| / 7\'7   Xilinx Spartan-XL I/O Buffer IBIS File
| \ \   Xilinx Inc.
| / /   2100 Logic Drive
| \_\/.\   San Jose,   CA 95124
[IBIS ver]   2.1
[File name]   xcs00xl.ibs
[File Rev]   2.1
[Date]   June 17, 1999
[Source]   Spice netlist
[Notes]   - Best/worse process data included in this ibis model
   - Control flag setting:
   SLW=0 - fast slew rate
   SLW=1 - slow slew rate
   PCI=0 - driving 3.3V PCI bus, 12mA
   PCI=1 - driving 5.0V PCI bus, 24mA
   5VT=0 - 5.0V tolerant input off
   5VT=1 - 5.0V tolerant input on
   - Created by Joey Jia x4437
[Copyright]   Xilinx Inc. All right reserved
|   Component XCS05XL_PC84[SLW=0;PCI=0;5VT=0]
[Component]   XCS05XL_PC84[SLW=0;PCI=0;5VT=0]
[Manufacturer]   Xilinx Inc.
[Package]
| variable   typ   min   max
R_pkg   0.104   97.000m   0.111
L_pkg   11.600nH   10.200nH   13.000nH
C_pkg   1.700pF   1.600pF   1.800pF
[Pin]  signal_name   model_name   R_pin   L_pin   C_pin
io   iob   IO_000   NA   NA   NA
|   Component XCS05XL_PC84[SLW=0;PCI=0;5VT=1]
[Component]   XCS05XL_PC84[SLW=0;PCI=0;5VT=1]
[Manufacturer]   Xilinx Inc.
[Package]
| variable   typ   min   max
R_pkg   0.104   97.000m   0.111
L_pkg   11.600nH   10.200nH   13.000nH
C_pkg   1.700pF   1.600pF   1.800pF
[Pin]  signal_name   model_name   R_pin   L_pin   C_pin
io   iob   IO_001   NA   NA   NA
|   Component XCS05XL_PC84[SLW=0;PCI=1;5VT=0]
[Component]   XCS05XL_PC84[SLW=0;PCI=1;5VT=0]
[Manufacturer]   Xilinx Inc.
[Package]
| variable   typ   min   max
R_pkg   0.104   97.000m   0.111
L_pkg   11.600nH   10.200nH   13.000nH
C_pkg   1.700pF   1.600pF   1.800pF
[Pin]  signal_name   model_name   R_pin   L_pin   C_pin
io   iob   IO_010   NA   NA   NA
|   Component XCS05XL_PC84[SLW=0;PCI=1;5VT=1]
[Component]   XCS05XL_PC84[SLW=0;PCI=1;5VT=1]
[Manufacturer]   Xilinx Inc.
[Package]
| variable   typ   min   max
R_pkg   0.104   97.000m   0.111
L_pkg   11.600nH   10.200nH   13.000nH
C_pkg   1.700pF   1.600pF   1.800pF
[Pin]  signal_name   model_name   R_pin   L_pin   C_pin
io   iob   IO_011   NA   NA   NA
|   Component XCS05XL_PC84[SLW=1;PCI=0;5VT=0]
[Component]   XCS05XL_PC84[SLW=1;PCI=0;5VT=0]
[Manufacturer]   Xilinx Inc.
[Package]
| variable   typ   min   max
R_pkg   0.104   97.000m   0.111
L_pkg   11.600nH   10.200nH   13.000nH
C_pkg   1.700pF   1.600pF   1.800pF
[Pin]  signal_name   model_name   R_pin   L_pin   C_pin
io   iob   IO_100   NA   NA   NA
|   Component XCS05XL_PC84[SLW=1;PCI=0;5VT=1]
[Component]   XCS05XL_PC84[SLW=1;PCI=0;5VT=1]
[Manufacturer]   Xilinx Inc.
[Package]
| variable   typ   min   max
R_pkg   0.104   97.000m   0.111
L_pkg   11.600nH   10.200nH   13.000nH
C_pkg   1.700pF   1.600pF   1.800pF
[Pin]  signal_name   model_name   R_pin   L_pin   C_pin
io   iob   IO_101   NA   NA   NA
|   Component XCS05XL_PC84[SLW=1;PCI=1;5VT=0]
[Component]   XCS05XL_PC84[SLW=1;PCI=1;5VT=0]
[Manufacturer]   Xilinx Inc.
[Package]
| variable   typ   min   max
R_pkg   0.104   97.000m   0.111
L_pkg   11.600nH   10.200nH   13.000nH
C_pkg   1.700pF   1.600pF   1.800pF
[Pin]  signal_name   model_name   R_pin   L_pin   C_pin
io   iob   IO_110   NA   NA   NA
|   Component XCS05XL_PC84[SLW=1;PCI=1;5VT=1]
[Component]   XCS05XL_PC84[SLW=1;PCI=1;5VT=1]
[Manufacturer]   Xilinx Inc.
[Package]
| variable   typ   min   max
R_pkg   0.104   97.000m   0.111
L_pkg   11.600nH   10.200nH   13.000nH
C_pkg   1.700pF   1.600pF   1.800pF
[Pin]  signal_name   model_name   R_pin   L_pin   C_pin
io   iob   IO_111   NA   NA   NA
|+++++++++++++++++++++++++++++++++++++++++++++++++++++++++++++++++++++++++
|   Component XCS05XL_VQ100[SLW=0;PCI=0;5VT=0]
[Component]   XCS05XL_VQ100[SLW=0;PCI=0;5VT=0]
[Manufacturer]   Xilinx Inc.
[Package]
| variable   typ   min   max
R_pkg   101.500m   98.000m   105.000m
L_pkg   5.200nH   4.700nH   5.700nH
C_pkg   0.550pF   0.400pF   0.700pF
[Pin]  signal_name   model_name   R_pin   L_pin   C_pin
io   iob   IO_000   NA   NA   NA
| End [Component] XCS05XL_VQ100[SLW=0;PCI=0;5VT=0]
|   Component XCS05XL_VQ100[SLW=0;PCI=0;5VT=1]
[Component]   XCS05XL_VQ100[SLW=0;PCI=0;5VT=1]
[Manufacturer]   Xilinx Inc.
[Package]
| variable   typ   min   max
R_pkg   101.500m   98.000m   105.000m
L_pkg   5.200nH   4.700nH   5.700nH
C_pkg   0.550pF   0.400pF   0.700pF
[Pin]  signal_name   model_name   R_pin   L_pin   C_pin
io   iob   IO_001   NA   NA   NA
| End [Component] XCS05XL_VQ100[SLW=0;PCI=0;5VT=1]
|   Component XCS05XL_VQ100[SLW=0;PCI=1;5VT=0]
[Component]   XCS05XL_VQ100[SLW=0;PCI=1;5VT=0]
[Manufacturer]   Xilinx Inc.
[Package]
| variable   typ   min   max
R_pkg   101.500m   98.000m   105.000m
L_pkg   5.200nH   4.700nH   5.700nH
C_pkg   0.550pF   0.400pF   0.700pF
[Pin]  signal_name   model_name   R_pin   L_pin   C_pin
io   iob   IO_010   NA   NA   NA
| End [Component] XCS05XL_VQ100[SLW=0;PCI=1;5VT=0]
|   Component XCS05XL_VQ100[SLW=0;PCI=1;5VT=1]
[Component]   XCS05XL_VQ100[SLW=0;PCI=1;5VT=1]
[Manufacturer]   Xilinx Inc.
[Package]
| variable   typ   min   max
R_pkg   101.500m   98.000m   105.000m
L_pkg   5.200nH   4.700nH   5.700nH
C_pkg   0.550pF   0.400pF   0.700pF
[Pin]  signal_name   model_name   R_pin   L_pin   C_pin
io   iob   IO_011   NA   NA   NA
| End [Component] XCS05XL_VQ100[SLW=0;PCI=1;5VT=1]
|   Component XCS05XL_VQ100[SLW=1;PCI=0;5VT=0]
[Component]   XCS05XL_VQ100[SLW=1;PCI=0;5VT=0]
[Manufacturer]   Xilinx Inc.
[Package]
| variable   typ   min   max
R_pkg   101.500m   98.000m   105.000m
L_pkg   5.200nH   4.700nH   5.700nH
C_pkg   0.550pF   0.400pF   0.700pF
[Pin]  signal_name   model_name   R_pin   L_pin   C_pin
io   iob   IO_100   NA   NA   NA
| End [Component] XCS05XL_VQ100[SLW=1;PCI=0;5VT=0]
|   Component XCS05XL_VQ101[SLW=1;PCI=0;5VT=1]
[Component]   XCS05XL_VQ100[SLW=1;PCI=0;5VT=1]
[Manufacturer]   Xilinx Inc.
[Package]
| variable   typ   min   max
R_pkg   101.500m   98.000m   105.000m
L_pkg   5.200nH   4.700nH   5.700nH
C_pkg   0.550pF   0.400pF   0.700pF
[Pin]  signal_name   model_name   R_pin   L_pin   C_pin
io   iob   IO_101   NA   NA   NA
| End [Component] XCS05XL_VQ100[SLW=1;PCI=0;5VT=1]
|   Component XCS05XL_VQ100[SLW=1;PCI=1;5VT=0]
[Component]   XCS05XL_VQ100[SLW=1;PCI=1;5VT=0]
[Manufacturer]   Xilinx Inc.
[Package]
| variable   typ   min   max
R_pkg   101.500m   98.000m   105.000m
L_pkg   5.200nH   4.700nH   5.700nH
C_pkg   0.550pF   0.400pF   0.700pF
[Pin]  signal_name   model_name   R_pin   L_pin   C_pin
io   iob   IO_110   NA   NA   NA
| End [Component] XCS05XL_VQ100[SLW=1;PCI=1;5VT=0]
|   Component XCS05XL_VQ100[SLW=1;PCI=1;5VT=1]
[Component]   XCS05XL_VQ100[SLW=1;PCI=1;5VT=1]
[Manufacturer]   Xilinx Inc.
[Package]
| variable   typ   min   max
R_pkg   101.500m   98.000m   105.000m
L_pkg   5.200nH   4.700nH   5.700nH
C_pkg   0.550pF   0.400pF   0.700pF
[Pin]  signal_name   model_name   R_pin   L_pin   C_pin
io   iob   IO_111   NA   NA   NA
| End [Component] XCS05XL_VQ100[SLW=1;PCI=1;5VT=1]
|+++++++++++++++++++++++++++++++++++++++++++++++++++++++++++++++++++++++++
|   Component XCS10XL_PC84[SLW=0;PCI=0;5VT=0]
[Component]   XCS10XL_PC84[SLW=0;PCI=0;5VT=0]
[Manufacturer]   Xilinx Inc.
[Package]
| variable   typ   min   max
R_pkg   104.000m   97.000m   111.000m
L_pkg   11.600nH   10.200nH   13.000nH
C_pkg   1.700pF   1.600pF   1.800pF
[Pin]  signal_name   model_name   R_pin   L_pin   C_pin
io   iob   IO_000   NA   NA   NA
| End [Component] XCS10XL_PC84[SLW=0;PCI=0;5VT=0]
|   Component XCS10XL_PC84[SLW=0;PCI=0;5VT=1]
[Component]   XCS10XL_PC84[SLW=0;PCI=0;5VT=1]
[Manufacturer]   Xilinx Inc.
[Package]
| variable   typ   min   max
R_pkg   104.000m   97.000m   111.000m
L_pkg   11.600nH   10.200nH   13.000nH
C_pkg   1.700pF   1.600pF   1.800pF
[Pin]  signal_name   model_name   R_pin   L_pin   C_pin
io   iob   IO_001   NA   NA   NA
| End [Component] XCS10XL_PC84[SLW=0;PCI=0;5VT=1]
|   Component XCS10XL_PC84[SLW=0;PCI=1;5VT=0]
[Component]   XCS10XL_PC84[SLW=0;PCI=1;5VT=0]
[Manufacturer]   Xilinx Inc.
[Package]
| variable   typ   min   max
R_pkg   104.000m   97.000m   111.000m
L_pkg   11.600nH   10.200nH   13.000nH
C_pkg   1.700pF   1.600pF   1.800pF
[Pin]  signal_name   model_name   R_pin   L_pin   C_pin
io   iob   IO_010   NA   NA   NA
| End [Component] XCS10XL_PC84[SLW=0;PCI=1;5VT=0]
|   Component XCS10XL_PC84[SLW=0;PCI=1;5VT=1]
[Component]   XCS10XL_PC84[SLW=0;PCI=1;5VT=1]
[Manufacturer]   Xilinx Inc.
[Package]
| variable   typ   min   max
R_pkg   104.000m   97.000m   111.000m
L_pkg   11.600nH   10.200nH   13.000nH
C_pkg   1.700pF   1.600pF   1.800pF
[Pin]  signal_name   model_name   R_pin   L_pin   C_pin
io   iob   IO_011   NA   NA   NA
| End [Component] XCS10XL_PC84[SLW=0;PCI=1;5VT=1]
|   Component XCS10XL_PC84[SLW=1;PCI=0;5VT=0]
[Component]   XCS10XL_PC84[SLW=1;PCI=0;5VT=0]
[Manufacturer]   Xilinx Inc.
[Package]
| variable   typ   min   max
R_pkg   104.000m   97.000m   111.000m
L_pkg   11.600nH   10.200nH   13.000nH
C_pkg   1.700pF   1.600pF   1.800pF
[Pin]  signal_name   model_name   R_pin   L_pin   C_pin
io   iob   IO_100   NA   NA   NA
| End [Component] XCS10XL_PC84[SLW=1;PCI=0;5VT=0]
|   Component XCS10XL_PC84[SLW=1;PCI=0;5VT=1]
[Component]   XCS10XL_PC84[SLW=1;PCI=0;5VT=1]
[Manufacturer]   Xilinx Inc.
[Package]
| variable   typ   min   max
R_pkg   104.000m   97.000m   111.000m
L_pkg   11.600nH   10.200nH   13.000nH
C_pkg   1.700pF   1.600pF   1.800pF
[Pin]  signal_name   model_name   R_pin   L_pin   C_pin
io   iob   IO_101   NA   NA   NA
| End [Component] XCS10XL_PC84[SLW=1;PCI=0;5VT=1]
|   Component XCS10XL_PC84[SLW=1;PCI=1;5VT=0]
[Component]   XCS10XL_PC84[SLW=1;PCI=1;5VT=0]
[Manufacturer]   Xilinx Inc.
[Package]
| variable   typ   min   max
R_pkg   104.000m   97.000m   111.000m
L_pkg   11.600nH   10.200nH   13.000nH
C_pkg   1.700pF   1.600pF   1.800pF
[Pin]  signal_name   model_name   R_pin   L_pin   C_pin
io   iob   IO_110   NA   NA   NA
| End [Component] XCS10XL_PC84[SLW=1;PCI=1;5VT=0]
|   Component XCS10XL_PC84[SLW=1;PCI=1;5VT=1]
[Component]   XCS10XL_PC84[SLW=1;PCI=1;5VT=1]
[Manufacturer]   Xilinx Inc.
[Package]
| variable   typ   min   max
R_pkg   104.000m   97.000m   111.000m
L_pkg   11.600nH   10.200nH   13.000nH
C_pkg   1.700pF   1.600pF   1.800pF
[Pin]  signal_name   model_name   R_pin   L_pin   C_pin
io   iob   IO_111   NA   NA   NA
| End [Component] XCS10XL_PC84[SLW=1;PCI=1;5VT=1]
|+++++++++++++++++++++++++++++++++++++++++++++++++++++++++++++++++++++++++
|   Component XCS10XL_VQ100[SLW=0;PCI=0;5VT=0]
[Component]   XCS10XL_VQ100[SLW=0;PCI=0;5VT=0]
[Manufacturer]   Xilinx Inc.
[Package]
| variable   typ   min   max
R_pkg   101.500m   98.000m   105.000m
L_pkg   5.200nH   4.700nH   5.700nH
C_pkg   0.550pF   0.400pF   0.700pF
[Pin]  signal_name   model_name   R_pin   L_pin   C_pin
io   iob   IO_000   NA   NA   NA
| End [Component] XCS10XL_VQ100[SLW=0;PCI=0;5VT=0]
|   Component XCS10XL_VQ100[SLW=0;PCI=0;5VT=1]
[Component]   XCS10XL_VQ100[SLW=0;PCI=0;5VT=1]
[Manufacturer]   Xilinx Inc.
[Package]
| variable   typ   min   max
R_pkg   101.500m   98.000m   105.000m
L_pkg   5.200nH   4.700nH   5.700nH
C_pkg   0.550pF   0.400pF   0.700pF
[Pin]  signal_name   model_name   R_pin   L_pin   C_pin
io   iob   IO_001   NA   NA   NA
| End [Component] XCS10XL_VQ100[SLW=0;PCI=0;5VT=1]
|   Component XCS10XL_VQ100[SLW=0;PCI=1;5VT=0]
[Component]   XCS10XL_VQ100[SLW=0;PCI=1;5VT=0]
[Manufacturer]   Xilinx Inc.
[Package]
| variable   typ   min   max
R_pkg   101.500m   98.000m   105.000m
L_pkg   5.200nH   4.700nH   5.700nH
C_pkg   0.550pF   0.400pF   0.700pF
[Pin]  signal_name   model_name   R_pin   L_pin   C_pin
io   iob   IO_010   NA   NA   NA
| End [Component] XCS10XL_VQ100[SLW=0;PCI=1;5VT=0]
|   Component XCS10XL_VQ100[SLW=0;PCI=1;5VT=1]
[Component]   XCS10XL_VQ100[SLW=0;PCI=1;5VT=1]
[Manufacturer]   Xilinx Inc.
[Package]
| variable   typ   min   max
R_pkg   101.500m   98.000m   105.000m
L_pkg   5.200nH   4.700nH   5.700nH
C_pkg   0.550pF   0.400pF   0.700pF
[Pin]  signal_name   model_name   R_pin   L_pin   C_pin
io   iob   IO_011   NA   NA   NA
| End [Component] XCS10XL_VQ100[SLW=0;PCI=1;5VT=1]
|   Component XCS10XL_VQ100[SLW=1;PCI=0;5VT=0]
[Component]   XCS10XL_VQ100[SLW=1;PCI=0;5VT=0]
[Manufacturer]   Xilinx Inc.
[Package]
| variable   typ   min   max
R_pkg   101.500m   98.000m   105.000m
L_pkg   5.200nH   4.700nH   5.700nH
C_pkg   0.550pF   0.400pF   0.700pF
[Pin]  signal_name   model_name   R_pin   L_pin   C_pin
io   iob   IO_100   NA   NA   NA
| End [Component] XCS10XL_VQ100[SLW=1;PCI=0;5VT=0]
|   Component XCS10XL_VQ100[SLW=1;PCI=0;5VT=1]
[Component]   XCS10XL_VQ100[SLW=1;PCI=0;5VT=1]
[Manufacturer]   Xilinx Inc.
[Package]
| variable   typ   min   max
R_pkg   101.500m   98.000m   105.000m
L_pkg   5.200nH   4.700nH   5.700nH
C_pkg   0.550pF   0.400pF   0.700pF
[Pin]  signal_name   model_name   R_pin   L_pin   C_pin
io   iob   IO_101   NA   NA   NA
| End [Component] XCS10XL_VQ100[SLW=1;PCI=0;5VT=1]
|   Component XCS10XL_VQ100[SLW=1;PCI=1;5VT=0]
[Component]   XCS10XL_VQ100[SLW=1;PCI=1;5VT=0]
[Manufacturer]   Xilinx Inc.
[Package]
| variable   typ   min   max
R_pkg   101.500m   98.000m   105.000m
L_pkg   5.200nH   4.700nH   5.700nH
C_pkg   0.550pF   0.400pF   0.700pF
[Pin]  signal_name   model_name   R_pin   L_pin   C_pin
io   iob   IO_110   NA   NA   NA
| End [Component] XCS10XL_VQ100[SLW=1;PCI=1;5VT=0]
|   Component XCS10XL_VQ100[SLW=1;PCI=1;5VT=1]
[Component]   XCS10XL_VQ100[SLW=1;PCI=1;5VT=1]
[Manufacturer]   Xilinx Inc.
[Package]
| variable   typ   min   max
R_pkg   101.500m   98.000m   105.000m
L_pkg   5.200nH   4.700nH   5.700nH
C_pkg   0.550pF   0.400pF   0.700pF
[Pin]  signal_name   model_name   R_pin   L_pin   C_pin
io   iob   IO_111   NA   NA   NA
| End [Component] XCS10XL_VQ100[SLW=1;PCI=1;5VT=1]
|+++++++++++++++++++++++++++++++++++++++++++++++++++++++++++++++++++++++++
|   Component XCS10XL_TQ144[SLW=0;PCI=0;5VT=0]
[Component]   XCS10XL_TQ144[SLW=0;PCI=0;5VT=0]
[Manufacturer]   Xilinx Inc.
[Package]
| variable   typ   min   max
R_pkg   123.500m   117.000m   130.000m
L_pkg   7.950nH   7.100nH   8.800nH
C_pkg   1.000pF   0.800pF   1.200pF
[Pin]  signal_name   model_name   R_pin   L_pin   C_pin
io   iob   IO_000   NA   NA   NA
| End [Component] XCS10XL_TQ144[SLW=0;PCI=0;5VT=0]
|   Component XCS10XL_TQ144[SLW=0;PCI=0;5VT=1]
[Component]   XCS10XL_TQ144[SLW=0;PCI=0;5VT=1]
[Manufacturer]   Xilinx Inc.
[Package]
| variable   typ   min   max
R_pkg   123.500m   117.000m   130.000m
L_pkg   7.950nH   7.100nH   8.800nH
C_pkg   1.000pF   0.800pF   1.200pF
[Pin]  signal_name   model_name   R_pin   L_pin   C_pin
io   iob   IO_001   NA   NA   NA
| End [Component] XCS10XL_TQ144[SLW=0;PCI=0;5VT=1]
|   Component XCS10XL_TQ144[SLW=0;PCI=1;5VT=0]
[Component]   XCS10XL_TQ144[SLW=0;PCI=1;5VT=0]
[Manufacturer]   Xilinx Inc.
[Package]
| variable   typ   min   max
R_pkg   123.500m   117.000m   130.000m
L_pkg   7.950nH   7.100nH   8.800nH
C_pkg   1.000pF   0.800pF   1.200pF
[Pin]  signal_name   model_name   R_pin   L_pin   C_pin
io   iob   IO_010   NA   NA   NA
| End [Component] XCS10XL_TQ144[SLW=0;PCI=1;5VT=0]
|   Component XCS10XL_TQ144[SLW=0;PCI=1;5VT=1]
[Component]   XCS10XL_TQ144[SLW=0;PCI=1;5VT=1]
[Manufacturer]   Xilinx Inc.
[Package]
| variable   typ   min   max
R_pkg   123.500m   117.000m   130.000m
L_pkg   7.950nH   7.100nH   8.800nH
C_pkg   1.000pF   0.800pF   1.200pF
[Pin]  signal_name   model_name   R_pin   L_pin   C_pin
io   iob   IO_011   NA   NA   NA
| End [Component] XCS10XL_TQ144[SLW=0;PCI=1;5VT=1]
|   Component XCS10XL_TQ144[SLW=1;PCI=0;5VT=0]
[Component]   XCS10XL_TQ144[SLW=1;PCI=0;5VT=0]
[Manufacturer]   Xilinx Inc.
[Package]
| variable   typ   min   max
R_pkg   123.500m   117.000m   130.000m
L_pkg   7.950nH   7.100nH   8.800nH
C_pkg   1.000pF   0.800pF   1.200pF
[Pin]  signal_name   model_name   R_pin   L_pin   C_pin
io   iob   IO_100   NA   NA   NA
| End [Component] XCS10XL_TQ144[SLW=1;PCI=0;5VT=0]
|   Component XCS10XL_TQ144[SLW=1;PCI=0;5VT=1]
[Component]   XCS10XL_TQ144[SLW=1;PCI=0;5VT=1]
[Manufacturer]   Xilinx Inc.
[Package]
| variable   typ   min   max
R_pkg   123.500m   117.000m   130.000m
L_pkg   7.950nH   7.100nH   8.800nH
C_pkg   1.000pF   0.800pF   1.200pF
[Pin]  signal_name   model_name   R_pin   L_pin   C_pin
io   iob   IO_101   NA   NA   NA
| End [Component] XCS10XL_TQ144[SLW=1;PCI=0;5VT=1]
|   Component XCS10XL_TQ144[SLW=1;PCI=1;5VT=0]
[Component]   XCS10XL_TQ144[SLW=1;PCI=1;5VT=0]
[Manufacturer]   Xilinx Inc.
[Package]
| variable   typ   min   max
R_pkg   123.500m   117.000m   130.000m
L_pkg   7.950nH   7.100nH   8.800nH
C_pkg   1.000pF   0.800pF   1.200pF
[Pin]  signal_name   model_name   R_pin   L_pin   C_pin
io   iob   IO_110   NA   NA   NA
| End [Component] XCS10XL_TQ144[SLW=1;PCI=1;5VT=0]
|   Component XCS10XL_TQ144[SLW=1;PCI=1;5VT=1]
[Component]   XCS10XL_TQ144[SLW=1;PCI=1;5VT=1]
[Manufacturer]   Xilinx Inc.
[Package]
| variable   typ   min   max
R_pkg   123.500m   117.000m   130.000m
L_pkg   7.950nH   7.100nH   8.800nH
C_pkg   1.000pF   0.800pF   1.200pF
[Pin]  signal_name   model_name   R_pin   L_pin   C_pin
io   iob   IO_111   NA   NA   NA
| End [Component] XCS10XL_TQ144[SLW=1;PCI=1;5VT=1]
|+++++++++++++++++++++++++++++++++++++++++++++++++++++++++++++++++++++++++
|   Component XCS20XL_VQ100[SLW=0;PCI=0;5VT=0]
[Component]   XCS20XL_VQ100[SLW=0;PCI=0;5VT=0]
[Manufacturer]   Xilinx Inc.
[Package]
| variable   typ   min   max
R_pkg   101.500m   98.000m   105.000m
L_pkg   5.200nH   4.700nH   5.700nH
C_pkg   0.550pF   0.400pF   0.700pF
[Pin]  signal_name   model_name   R_pin   L_pin   C_pin
io   iob   IO_000   NA   NA   NA
| End [Component] XCS20XL_VQ100[SLW=0;PCI=0;5VT=0]
|   Component XCS20XL_VQ100[SLW=0;PCI=0;5VT=1]
[Component]   XCS20XL_VQ100[SLW=0;PCI=0;5VT=1]
[Manufacturer]   Xilinx Inc.
[Package]
| variable   typ   min   max
R_pkg   101.500m   98.000m   105.000m
L_pkg   5.200nH   4.700nH   5.700nH
C_pkg   0.550pF   0.400pF   0.700pF
[Pin]  signal_name   model_name   R_pin   L_pin   C_pin
io   iob   IO_001   NA   NA   NA
| End [Component] XCS20XL_VQ100[SLW=0;PCI=0;5VT=1]
|   Component XCS20XL_VQ100[SLW=0;PCI=1;5VT=0]
[Component]   XCS20XL_VQ100[SLW=0;PCI=1;5VT=0]
[Manufacturer]   Xilinx Inc.
[Package]
| variable   typ   min   max
R_pkg   101.500m   98.000m   105.000m
L_pkg   5.200nH   4.700nH   5.700nH
C_pkg   0.550pF   0.400pF   0.700pF
[Pin]  signal_name   model_name   R_pin   L_pin   C_pin
io   iob   IO_010   NA   NA   NA
| End [Component] XCS20XL_VQ100[SLW=0;PCI=1;5VT=0]
|   Component XCS20XL_VQ100[SLW=0;PCI=1;5VT=1]
[Component]   XCS20XL_VQ100[SLW=0;PCI=1;5VT=1]
[Manufacturer]   Xilinx Inc.
[Package]
| variable   typ   min   max
R_pkg   101.500m   98.000m   105.000m
L_pkg   5.200nH   4.700nH   5.700nH
C_pkg   0.550pF   0.400pF   0.700pF
[Pin]  signal_name   model_name   R_pin   L_pin   C_pin
io   iob   IO_011   NA   NA   NA
| End [Component] XCS20XL_VQ100[SLW=0;PCI=1;5VT=1]
|   Component XCS20XL_VQ100[SLW=1;PCI=0;5VT=0]
[Component]   XCS20XL_VQ100[SLW=1;PCI=0;5VT=0]
[Manufacturer]   Xilinx Inc.
[Package]
| variable   typ   min   max
R_pkg   101.500m   98.000m   105.000m
L_pkg   5.200nH   4.700nH   5.700nH
C_pkg   0.550pF   0.400pF   0.700pF
[Pin]  signal_name   model_name   R_pin   L_pin   C_pin
io   iob   IO_100   NA   NA   NA
| End [Component] XCS20XL_VQ100[SLW=1;PCI=0;5VT=0]
|   Component XCS20XL_VQ100[SLW=1;PCI=0;5VT=1]
[Component]   XCS20XL_VQ100[SLW=1;PCI=0;5VT=1]
[Manufacturer]   Xilinx Inc.
[Package]
| variable   typ   min   max
R_pkg   101.500m   98.000m   105.000m
L_pkg   5.200nH   4.700nH   5.700nH
C_pkg   0.550pF   0.400pF   0.700pF
[Pin]  signal_name   model_name   R_pin   L_pin   C_pin
io   iob   IO_101   NA   NA   NA
| End [Component] XCS20XL_VQ100[SLW=1;PCI=0;5VT=1]
|   Component XCS20XL_VQ100[SLW=1;PCI=1;5VT=0]
[Component]   XCS20XL_VQ100[SLW=1;PCI=1;5VT=0]
[Manufacturer]   Xilinx Inc.
[Package]
| variable   typ   min   max
R_pkg   101.500m   98.000m   105.000m
L_pkg   5.200nH   4.700nH   5.700nH
C_pkg   0.550pF   0.400pF   0.700pF
[Pin]  signal_name   model_name   R_pin   L_pin   C_pin
io   iob   IO_110   NA   NA   NA
| End [Component] XCS20XL_VQ100[SLW=1;PCI=1;5VT=0]
|   Component XCS20XL_VQ100[SLW=1;PCI=1;5VT=1]
[Component]   XCS20XL_VQ100[SLW=1;PCI=1;5VT=1]
[Manufacturer]   Xilinx Inc.
[Package]
| variable   typ   min   max
R_pkg   101.500m   98.000m   105.000m
L_pkg   5.200nH   4.700nH   5.700nH
C_pkg   0.550pF   0.400pF   0.700pF
[Pin]  signal_name   model_name   R_pin   L_pin   C_pin
io   iob   IO_111   NA   NA   NA
| End [Component] XCS20XL_VQ100[SLW=1;PCI=1;5VT=1]
|+++++++++++++++++++++++++++++++++++++++++++++++++++++++++++++++++++++++++
|   Component XCS20XL_TQ144[SLW=0;PCI=0;5VT=0]
[Component]   XCS20XL_TQ144[SLW=0;PCI=0;5VT=0]
[Manufacturer]   Xilinx Inc.
[Package]
| variable   typ   min   max
R_pkg   123.500m   117.000m   130.000m
L_pkg   7.950nH   7.100nH   8.800nH
C_pkg   1.000pF   0.800pF   1.200pF
[Pin]  signal_name   model_name   R_pin   L_pin   C_pin
io   iob   IO_000   NA   NA   NA
| End [Component] XCS20XL_TQ144[SLW=0;PCI=0;5VT=0]
|   Component XCS20XL_TQ144[SLW=0;PCI=0;5VT=1]
[Component]   XCS20XL_TQ144[SLW=0;PCI=0;5VT=1]
[Manufacturer]   Xilinx Inc.
[Package]
| variable   typ   min   max
R_pkg   123.500m   117.000m   130.000m
L_pkg   7.950nH   7.100nH   8.800nH
C_pkg   1.000pF   0.800pF   1.200pF
[Pin]  signal_name   model_name   R_pin   L_pin   C_pin
io   iob   IO_001   NA   NA   NA
| End [Component] XCS20XL_TQ144[SLW=0;PCI=0;5VT=1]
|   Component XCS20XL_TQ144[SLW=0;PCI=1;5VT=0]
[Component]   XCS20XL_TQ144[SLW=0;PCI=1;5VT=0]
[Manufacturer]   Xilinx Inc.
[Package]
| variable   typ   min   max
R_pkg   123.500m   117.000m   130.000m
L_pkg   7.950nH   7.100nH   8.800nH
C_pkg   1.000pF   0.800pF   1.200pF
[Pin]  signal_name   model_name   R_pin   L_pin   C_pin
io   iob   IO_010   NA   NA   NA
| End [Component] XCS20XL_TQ144[SLW=0;PCI=1;5VT=0]
|   Component XCS20XL_TQ144[SLW=0;PCI=1;5VT=1]
[Component]   XCS20XL_TQ144[SLW=0;PCI=1;5VT=1]
[Manufacturer]   Xilinx Inc.
[Package]
| variable   typ   min   max
R_pkg   123.500m   117.000m   130.000m
L_pkg   7.950nH   7.100nH   8.800nH
C_pkg   1.000pF   0.800pF   1.200pF
[Pin]  signal_name   model_name   R_pin   L_pin   C_pin
io   iob   IO_011   NA   NA   NA
| End [Component] XCS20XL_TQ144[SLW=0;PCI=1;5VT=1]
|   Component XCS20XL_TQ144[SLW=1;PCI=0;5VT=0]
[Component]   XCS20XL_TQ144[SLW=1;PCI=0;5VT=0]
[Manufacturer]   Xilinx Inc.
[Package]
| variable   typ   min   max
R_pkg   123.500m   117.000m   130.000m
L_pkg   7.950nH   7.100nH   8.800nH
C_pkg   1.000pF   0.800pF   1.200pF
[Pin]  signal_name   model_name   R_pin   L_pin   C_pin
io   iob   IO_100   NA   NA   NA
| End [Component] XCS20XL_TQ144[SLW=1;PCI=0;5VT=0]
|   Component XCS20XL_TQ144[SLW=1;PCI=0;5VT=1]
[Component]   XCS20XL_TQ144[SLW=1;PCI=0;5VT=1]
[Manufacturer]   Xilinx Inc.
[Package]
| variable   typ   min   max
R_pkg   123.500m   117.000m   130.000m
L_pkg   7.950nH   7.100nH   8.800nH
C_pkg   1.000pF   0.800pF   1.200pF
[Pin]  signal_name   model_name   R_pin   L_pin   C_pin
io   iob   IO_101   NA   NA   NA
| End [Component] XCS20XL_TQ144[SLW=1;PCI=0;5VT=1]
|   Component XCS20XL_TQ144[SLW=1;PCI=1;5VT=0]
[Component]   XCS20XL_TQ144[SLW=1;PCI=1;5VT=0]
[Manufacturer]   Xilinx Inc.
[Package]
| variable   typ   min   max
R_pkg   123.500m   117.000m   130.000m
L_pkg   7.950nH   7.100nH   8.800nH
C_pkg   1.000pF   0.800pF   1.200pF
[Pin]  signal_name   model_name   R_pin   L_pin   C_pin
io   iob   IO_110   NA   NA   NA
| End [Component] XCS20XL_TQ144[SLW=1;PCI=1;5VT=0]
|   Component XCS20XL_TQ144[SLW=1;PCI=1;5VT=1]
[Component]   XCS20XL_TQ144[SLW=1;PCI=1;5VT=1]
[Manufacturer]   Xilinx Inc.
[Package]
| variable   typ   min   max
R_pkg   123.500m   117.000m   130.000m
L_pkg   7.950nH   7.100nH   8.800nH
C_pkg   1.000pF   0.800pF   1.200pF
[Pin]  signal_name   model_name   R_pin   L_pin   C_pin
io   iob   IO_111   NA   NA   NA
| End [Component] XCS20XL_TQ144[SLW=1;PCI=1;5VT=1]
|+++++++++++++++++++++++++++++++++++++++++++++++++++++++++++++++++++++++++
|   Component XCS20XL_PQ208[SLW=0;PCI=0;5VT=0]
[Component]   XCS20XL_PQ208[SLW=0;PCI=0;5VT=0]
[Manufacturer]   Xilinx Inc.
[Package]
| variable   typ   min   max
R_pkg   195.500m   195.000m   196.000m
L_pkg   14.200nH   12.500nH   15.900nH
C_pkg   1.800pF   1.600pF   2.000pF
[Pin]  signal_name   model_name   R_pin   L_pin   C_pin
io   iob   IO_000   NA   NA   NA
| End [Component] XCS20XL_PQ208[SLW=0;PCI=0;5VT=0]
|   Component XCS20XL_PQ208[SLW=0;PCI=0;5VT=1]
[Component]   XCS20XL_PQ208[SLW=0;PCI=0;5VT=1]
[Manufacturer]   Xilinx Inc.
[Package]
| variable   typ   min   max
R_pkg   195.500m   195.000m   196.000m
L_pkg   14.200nH   12.500nH   15.900nH
C_pkg   1.800pF   1.600pF   2.000pF
[Pin]  signal_name   model_name   R_pin   L_pin   C_pin
io   iob   IO_001   NA   NA   NA
| End [Component] XCS20XL_PQ208[SLW=0;PCI=0;5VT=1]
|   Component XCS20XL_PQ208[SLW=0;PCI=1;5VT=0]
[Component]   XCS20XL_PQ208[SLW=0;PCI=1;5VT=0]
[Manufacturer]   Xilinx Inc.
[Package]
| variable   typ   min   max
R_pkg   195.500m   195.000m   196.000m
L_pkg   14.200nH   12.500nH   15.900nH
C_pkg   1.800pF   1.600pF   2.000pF
[Pin]  signal_name   model_name   R_pin   L_pin   C_pin
io   iob   IO_010   NA   NA   NA
| End [Component] XCS20XL_PQ208[SLW=0;PCI=1;5VT=0]
|   Component XCS20XL_PQ208[SLW=0;PCI=1;5VT=1]
[Component]   XCS20XL_PQ208[SLW=0;PCI=1;5VT=1]
[Manufacturer]   Xilinx Inc.
[Package]
| variable   typ   min   max
R_pkg   195.500m   195.000m   196.000m
L_pkg   14.200nH   12.500nH   15.900nH
C_pkg   1.800pF   1.600pF   2.000pF
[Pin]  signal_name   model_name   R_pin   L_pin   C_pin
io   iob   IO_011   NA   NA   NA
| End [Component] XCS20XL_PQ208[SLW=0;PCI=1;5VT=1]
|   Component XCS20XL_PQ208[SLW=1;PCI=0;5VT=0]
[Component]   XCS20XL_PQ208[SLW=1;PCI=0;5VT=0]
[Manufacturer]   Xilinx Inc.
[Package]
| variable   typ   min   max
R_pkg   195.500m   195.000m   196.000m
L_pkg   14.200nH   12.500nH   15.900nH
C_pkg   1.800pF   1.600pF   2.000pF
[Pin]  signal_name   model_name   R_pin   L_pin   C_pin
io   iob   IO_100   NA   NA   NA
| End [Component] XCS20XL_PQ208[SLW=1;PCI=0;5VT=0]
|   Component XCS20XL_PQ208[SLW=1;PCI=0;5VT=1]
[Component]   XCS20XL_PQ208[SLW=1;PCI=0;5VT=1]
[Manufacturer]   Xilinx Inc.
[Package]
| variable   typ   min   max
R_pkg   195.500m   195.000m   196.000m
L_pkg   14.200nH   12.500nH   15.900nH
C_pkg   1.800pF   1.600pF   2.000pF
[Pin]  signal_name   model_name   R_pin   L_pin   C_pin
io   iob   IO_101   NA   NA   NA
| End [Component] XCS20XL_PQ208[SLW=1;PCI=0;5VT=1]
|   Component XCS20XL_PQ208[SLW=1;PCI=1;5VT=0]
[Component]   XCS20XL_PQ208[SLW=1;PCI=1;5VT=0]
[Manufacturer]   Xilinx Inc.
[Package]
| variable   typ   min   max
R_pkg   195.500m   195.000m   196.000m
L_pkg   14.200nH   12.500nH   15.900nH
C_pkg   1.800pF   1.600pF   2.000pF
[Pin]  signal_name   model_name   R_pin   L_pin   C_pin
io   iob   IO_110   NA   NA   NA
| End [Component] XCS20XL_PQ208[SLW=1;PCI=1;5VT=0]
|   Component XCS20XL_PQ208[SLW=1;PCI=1;5VT=1]
[Component]   XCS20XL_PQ208[SLW=1;PCI=1;5VT=1]
[Manufacturer]   Xilinx Inc.
[Package]
| variable   typ   min   max
R_pkg   195.500m   195.000m   196.000m
L_pkg   14.200nH   12.500nH   15.900nH
C_pkg   1.800pF   1.600pF   2.000pF
[Pin]  signal_name   model_name   R_pin   L_pin   C_pin
io   iob   IO_111   NA   NA   NA
| End [Component] XCS20XL_PQ208[SLW=1;PCI=1;5VT=1]
|+++++++++++++++++++++++++++++++++++++++++++++++++++++++++++++++++++++++++
|   Component XCS30XL_VQ100[SLW=0;PCI=0;5VT=0]
[Component]   XCS30XL_VQ100[SLW=0;PCI=0;5VT=0]
[Manufacturer]   Xilinx Inc.
[Package]
| variable   typ   min   max
R_pkg   84.500m   79.000m   90.000m
L_pkg   4.350nH   3.800nH   4.900nH
C_pkg   0.650pF   0.600pF   0.700pF
[Pin]  signal_name   model_name   R_pin   L_pin   C_pin
io   iob   IO_000   NA   NA   NA
| End [Component] XCS30XL_VQ100[SLW=0;PCI=0;5VT=0]
|   Component XCS30XL_VQ100[SLW=0;PCI=0;5VT=1]
[Component]   XCS30XL_VQ100[SLW=0;PCI=0;5VT=1]
[Manufacturer]   Xilinx Inc.
[Package]
| variable   typ   min   max
R_pkg   84.500m   79.000m   90.000m
L_pkg   4.350nH   3.800nH   4.900nH
C_pkg   0.650pF   0.600pF   0.700pF
[Pin]  signal_name   model_name   R_pin   L_pin   C_pin
io   iob   IO_001   NA   NA   NA
| End [Component] XCS30XL_VQ100[SLW=0;PCI=0;5VT=1]
|   Component XCS30XL_VQ100[SLW=0;PCI=1;5VT=0]
[Component]   XCS30XL_VQ100[SLW=0;PCI=1;5VT=0]
[Manufacturer]   Xilinx Inc.
[Package]
| variable   typ   min   max
R_pkg   84.500m   79.000m   90.000m
L_pkg   4.350nH   3.800nH   4.900nH
C_pkg   0.650pF   0.600pF   0.700pF
[Pin]  signal_name   model_name   R_pin   L_pin   C_pin
io   iob   IO_010   NA   NA   NA
| End [Component] XCS30XL_VQ100[SLW=0;PCI=1;5VT=0]
|   Component XCS30XL_VQ100[SLW=0;PCI=1;5VT=1]
[Component]   XCS30XL_VQ100[SLW=0;PCI=1;5VT=1]
[Manufacturer]   Xilinx Inc.
[Package]
| variable   typ   min   max
R_pkg   84.500m   79.000m   90.000m
L_pkg   4.350nH   3.800nH   4.900nH
C_pkg   0.650pF   0.600pF   0.700pF
[Pin]  signal_name   model_name   R_pin   L_pin   C_pin
io   iob   IO_011   NA   NA   NA
| End [Component] XCS30XL_VQ100[SLW=0;PCI=1;5VT=1]
|   Component XCS30XL_VQ100[SLW=1;PCI=0;5VT=0]
[Component]   XCS30XL_VQ100[SLW=1;PCI=0;5VT=0]
[Manufacturer]   Xilinx Inc.
[Package]
| variable   typ   min   max
R_pkg   84.500m   79.000m   90.000m
L_pkg   4.350nH   3.800nH   4.900nH
C_pkg   0.650pF   0.600pF   0.700pF
[Pin]  signal_name   model_name   R_pin   L_pin   C_pin
io   iob   IO_100   NA   NA   NA
| End [Component] XCS30XL_VQ100[SLW=1;PCI=0;5VT=0]
|   Component XCS30XL_VQ100[SLW=1;PCI=0;5VT=1]
[Component]   XCS30XL_VQ100[SLW=1;PCI=0;5VT=1]
[Manufacturer]   Xilinx Inc.
[Package]
| variable   typ   min   max
R_pkg   84.500m   79.000m   90.000m
L_pkg   4.350nH   3.800nH   4.900nH
C_pkg   0.650pF   0.600pF   0.700pF
[Pin]  signal_name   model_name   R_pin   L_pin   C_pin
io   iob   IO_101   NA   NA   NA
| End [Component] XCS30XL_VQ100[SLW=1;PCI=0;5VT=1]
|   Component XCS30XL_VQ100[SLW=1;PCI=1;5VT=0]
[Component]   XCS30XL_VQ100[SLW=1;PCI=1;5VT=0]
[Manufacturer]   Xilinx Inc.
[Package]
| variable   typ   min   max
R_pkg   84.500m   79.000m   90.000m
L_pkg   4.350nH   3.800nH   4.900nH
C_pkg   0.650pF   0.600pF   0.700pF
[Pin]  signal_name   model_name   R_pin   L_pin   C_pin
io   iob   IO_110   NA   NA   NA
| End [Component] XCS30XL_VQ100[SLW=1;PCI=1;5VT=0]
|   Component XCS30XL_VQ100[SLW=1;PCI=1;5VT=1]
[Component]   XCS30XL_VQ100[SLW=1;PCI=1;5VT=1]
[Manufacturer]   Xilinx Inc.
[Package]
| variable   typ   min   max
R_pkg   84.500m   79.000m   90.000m
L_pkg   4.350nH   3.800nH   4.900nH
C_pkg   0.650pF   0.600pF   0.700pF
[Pin]  signal_name   model_name   R_pin   L_pin   C_pin
io   iob   IO_111   NA   NA   NA
| End [Component] XCS30XL_VQ100[SLW=1;PCI=1;5VT=1]
|+++++++++++++++++++++++++++++++++++++++++++++++++++++++++++++++++++++++++
|   Component XCS30XL_TQ144[SLW=0;PCI=0;5VT=0]
[Component]   XCS30XL_TQ144[SLW=0;PCI=0;5VT=0]
[Manufacturer]   Xilinx Inc.
[Package]
| variable   typ   min   max
R_pkg   123.500m   117.000m   130.000m
L_pkg   7.950nH   7.100nH   8.800nH
C_pkg   1.000pF   0.800pF   1.200pF
[Pin]  signal_name   model_name   R_pin   L_pin   C_pin
io   iob   IO_000   NA   NA   NA
| End [Component] XCS30XL_TQ144[SLW=0;PCI=0;5VT=0]
|   Component XCS30XL_TQ144[SLW=0;PCI=0;5VT=1]
[Component]   XCS30XL_TQ144[SLW=0;PCI=0;5VT=1]
[Manufacturer]   Xilinx Inc.
[Package]
| variable   typ   min   max
R_pkg   123.500m   117.000m   130.000m
L_pkg   7.950nH   7.100nH   8.800nH
C_pkg   1.000pF   0.800pF   1.200pF
[Pin]  signal_name   model_name   R_pin   L_pin   C_pin
io   iob   IO_001   NA   NA   NA
| End [Component] XCS30XL_TQ144[SLW=0;PCI=0;5VT=1]
|   Component XCS30XL_TQ144[SLW=0;PCI=1;5VT=0]
[Component]   XCS30XL_TQ144[SLW=0;PCI=1;5VT=0]
[Manufacturer]   Xilinx Inc.
[Package]
| variable   typ   min   max
R_pkg   123.500m   117.000m   130.000m
L_pkg   7.950nH   7.100nH   8.800nH
C_pkg   1.000pF   0.800pF   1.200pF
[Pin]  signal_name   model_name   R_pin   L_pin   C_pin
io   iob   IO_010   NA   NA   NA
| End [Component] XCS30XL_TQ144[SLW=0;PCI=1;5VT=0]
|   Component XCS30XL_TQ144[SLW=0;PCI=1;5VT=1]
[Component]   XCS30XL_TQ144[SLW=0;PCI=1;5VT=1]
[Manufacturer]   Xilinx Inc.
[Package]
| variable   typ   min   max
R_pkg   123.500m   117.000m   130.000m
L_pkg   7.950nH   7.100nH   8.800nH
C_pkg   1.000pF   0.800pF   1.200pF
[Pin]  signal_name   model_name   R_pin   L_pin   C_pin
io   iob   IO_011   NA   NA   NA
| End [Component] XCS30XL_TQ144[SLW=0;PCI=1;5VT=1]
|   Component XCS30XL_TQ144[SLW=1;PCI=0;5VT=0]
[Component]   XCS30XL_TQ144[SLW=1;PCI=0;5VT=0]
[Manufacturer]   Xilinx Inc.
[Package]
| variable   typ   min   max
R_pkg   123.500m   117.000m   130.000m
L_pkg   7.950nH   7.100nH   8.800nH
C_pkg   1.000pF   0.800pF   1.200pF
[Pin]  signal_name   model_name   R_pin   L_pin   C_pin
io   iob   IO_100   NA   NA   NA
| End [Component] XCS30XL_TQ144[SLW=1;PCI=0;5VT=0]
|   Component XCS30XL_TQ144[SLW=1;PCI=0;5VT=1]
[Component]   XCS30XL_TQ144[SLW=1;PCI=0;5VT=1]
[Manufacturer]   Xilinx Inc.
[Package]
| variable   typ   min   max
R_pkg   123.500m   117.000m   130.000m
L_pkg   7.950nH   7.100nH   8.800nH
C_pkg   1.000pF   0.800pF   1.200pF
[Pin]  signal_name   model_name   R_pin   L_pin   C_pin
io   iob   IO_101   NA   NA   NA
| End [Component] XCS30XL_TQ144[SLW=1;PCI=0;5VT=1]
|   Component XCS30XL_TQ144[SLW=1;PCI=1;5VT=0]
[Component]   XCS30XL_TQ144[SLW=1;PCI=1;5VT=0]
[Manufacturer]   Xilinx Inc.
[Package]
| variable   typ   min   max
R_pkg   123.500m   117.000m   130.000m
L_pkg   7.950nH   7.100nH   8.800nH
C_pkg   1.000pF   0.800pF   1.200pF
[Pin]  signal_name   model_name   R_pin   L_pin   C_pin
io   iob   IO_110   NA   NA   NA
| End [Component] XCS30XL_TQ144[SLW=1;PCI=1;5VT=0]
|   Component XCS30XL_TQ144[SLW=1;PCI=1;5VT=1]
[Component]   XCS30XL_TQ144[SLW=1;PCI=1;5VT=1]
[Manufacturer]   Xilinx Inc.
[Package]
| variable   typ   min   max
R_pkg   123.500m   117.000m   130.000m
L_pkg   7.950nH   7.100nH   8.800nH
C_pkg   1.000pF   0.800pF   1.200pF
[Pin]  signal_name   model_name   R_pin   L_pin   C_pin
io   iob   IO_111   NA   NA   NA
| End [Component] XCS30XL_TQ144[SLW=1;PCI=1;5VT=1]
|+++++++++++++++++++++++++++++++++++++++++++++++++++++++++++++++++++++++++
|   Component XCS30XL_PQ208[SLW=0;PCI=0;5VT=0]
[Component]   XCS30XL_PQ208[SLW=0;PCI=0;5VT=0]
[Manufacturer]   Xilinx Inc.
[Package]
| variable   typ   min   max
R_pkg   195.500m   195.000m   196.000m
L_pkg   14.200nH   12.500nH   15.900nH
C_pkg   1.800pF   1.600pF   2.000pF
[Pin]  signal_name   model_name   R_pin   L_pin   C_pin
io   iob   IO_000   NA   NA   NA
| End [Component] XCS30XL_PQ208[SLW=0;PCI=0;5VT=0]
|   Component XCS30XL_PQ208[SLW=0;PCI=0;5VT=1]
[Component]   XCS30XL_PQ208[SLW=0;PCI=0;5VT=1]
[Manufacturer]   Xilinx Inc.
[Package]
| variable   typ   min   max
R_pkg   195.500m   195.000m   196.000m
L_pkg   14.200nH   12.500nH   15.900nH
C_pkg   1.800pF   1.600pF   2.000pF
[Pin]  signal_name   model_name   R_pin   L_pin   C_pin
io   iob   IO_001   NA   NA   NA
| End [Component] XCS30XL_PQ208[SLW=0;PCI=0;5VT=1]
|   Component XCS30XL_PQ208[SLW=0;PCI=1;5VT=0]
[Component]   XCS30XL_PQ208[SLW=0;PCI=1;5VT=0]
[Manufacturer]   Xilinx Inc.
[Package]
| variable   typ   min   max
R_pkg   195.500m   195.000m   196.000m
L_pkg   14.200nH   12.500nH   15.900nH
C_pkg   1.800pF   1.600pF   2.000pF
[Pin]  signal_name   model_name   R_pin   L_pin   C_pin
io   iob   IO_010   NA   NA   NA
| End [Component] XCS30XL_PQ208[SLW=0;PCI=1;5VT=0]
|   Component XCS30XL_PQ208[SLW=0;PCI=1;5VT=1]
[Component]   XCS30XL_PQ208[SLW=0;PCI=1;5VT=1]
[Manufacturer]   Xilinx Inc.
[Package]
| variable   typ   min   max
R_pkg   195.500m   195.000m   196.000m
L_pkg   14.200nH   12.500nH   15.900nH
C_pkg   1.800pF   1.600pF   2.000pF
[Pin]  signal_name   model_name   R_pin   L_pin   C_pin
io   iob   IO_011   NA   NA   NA
| End [Component] XCS30XL_PQ208[SLW=0;PCI=1;5VT=1]
|   Component XCS30XL_PQ208[SLW=1;PCI=0;5VT=0]
[Component]   XCS30XL_PQ208[SLW=1;PCI=0;5VT=0]
[Manufacturer]   Xilinx Inc.
[Package]
| variable   typ   min   max
R_pkg   195.500m   195.000m   196.000m
L_pkg   14.200nH   12.500nH   15.900nH
C_pkg   1.800pF   1.600pF   2.000pF
[Pin]  signal_name   model_name   R_pin   L_pin   C_pin
io   iob   IO_100   NA   NA   NA
| End [Component] XCS30XL_PQ208[SLW=1;PCI=0;5VT=0]
|   Component XCS30XL_PQ208[SLW=1;PCI=0;5VT=1]
[Component]   XCS30XL_PQ208[SLW=1;PCI=0;5VT=1]
[Manufacturer]   Xilinx Inc.
[Package]
| variable   typ   min   max
R_pkg   195.500m   195.000m   196.000m
L_pkg   14.200nH   12.500nH   15.900nH
C_pkg   1.800pF   1.600pF   2.000pF
[Pin]  signal_name   model_name   R_pin   L_pin   C_pin
io   iob   IO_101   NA   NA   NA
| End [Component] XCS30XL_PQ208[SLW=1;PCI=0;5VT=1]
|   Component XCS30XL_PQ208[SLW=1;PCI=1;5VT=0]
[Component]   XCS30XL_PQ208[SLW=1;PCI=1;5VT=0]
[Manufacturer]   Xilinx Inc.
[Package]
| variable   typ   min   max
R_pkg   195.500m   195.000m   196.000m
L_pkg   14.200nH   12.500nH   15.900nH
C_pkg   1.800pF   1.600pF   2.000pF
[Pin]  signal_name   model_name   R_pin   L_pin   C_pin
io   iob   IO_110   NA   NA   NA
| End [Component] XCS30XL_PQ208[SLW=1;PCI=1;5VT=0]
|   Component XCS30XL_PQ208[SLW=1;PCI=1;5VT=1]
[Component]   XCS30XL_PQ208[SLW=1;PCI=1;5VT=1]
[Manufacturer]   Xilinx Inc.
[Package]
| variable   typ   min   max
R_pkg   195.500m   195.000m   196.000m
L_pkg   14.200nH   12.500nH   15.900nH
C_pkg   1.800pF   1.600pF   2.000pF
[Pin]  signal_name   model_name   R_pin   L_pin   C_pin
io   iob   IO_111   NA   NA   NA
| End [Component] XCS30XL_PQ208[SLW=1;PCI=1;5VT=1]
|+++++++++++++++++++++++++++++++++++++++++++++++++++++++++++++++++++++++++
|   Component XCS30XL_PQ240[SLW=0;PCI=0;5VT=0]
[Component]   XCS30XL_PQ240[SLW=0;PCI=0;5VT=0]
[Manufacturer]   Xilinx Inc.
[Package]
| variable   typ   min   max
R_pkg   211.500m   205.000m   218.000m
L_pkg   14.500nH   12.200nH   16.800nH
C_pkg   2.150pF   2.000pF   2.300pF
[Pin]  signal_name   model_name   R_pin   L_pin   C_pin
io   iob   IO_000   NA   NA   NA
| End [Component] XCS30XL_PQ240[SLW=0;PCI=0;5VT=0]
|   Component XCS30XL_PQ240[SLW=0;PCI=0;5VT=1]
[Component]   XCS30XL_PQ240[SLW=0;PCI=0;5VT=1]
[Manufacturer]   Xilinx Inc.
[Package]
| variable   typ   min   max
R_pkg   211.500m   205.000m   218.000m
L_pkg   14.500nH   12.200nH   16.800nH
C_pkg   2.150pF   2.000pF   2.300pF
[Pin]  signal_name   model_name   R_pin   L_pin   C_pin
io   iob   IO_001   NA   NA   NA
| End [Component] XCS30XL_PQ240[SLW=0;PCI=0;5VT=1]
|   Component XCS30XL_PQ240[SLW=0;PCI=1;5VT=0]
[Component]   XCS30XL_PQ240[SLW=0;PCI=1;5VT=0]
[Manufacturer]   Xilinx Inc.
[Package]
| variable   typ   min   max
R_pkg   211.500m   205.000m   218.000m
L_pkg   14.500nH   12.200nH   16.800nH
C_pkg   2.150pF   2.000pF   2.300pF
[Pin]  signal_name   model_name   R_pin   L_pin   C_pin
io   iob   IO_010   NA   NA   NA
| End [Component] XCS30XL_PQ240[SLW=0;PCI=1;5VT=0]
|   Component XCS30XL_PQ240[SLW=0;PCI=1;5VT=1]
[Component]   XCS30XL_PQ240[SLW=0;PCI=1;5VT=1]
[Manufacturer]   Xilinx Inc.
[Package]
| variable   typ   min   max
R_pkg   211.500m   205.000m   218.000m
L_pkg   14.500nH   12.200nH   16.800nH
C_pkg   2.150pF   2.000pF   2.300pF
[Pin]  signal_name   model_name   R_pin   L_pin   C_pin
io   iob   IO_011   NA   NA   NA
| End [Component] XCS30XL_PQ240[SLW=0;PCI=1;5VT=1]
|   Component XCS30XL_PQ240[SLW=1;PCI=0;5VT=0]
[Component]   XCS30XL_PQ240[SLW=1;PCI=0;5VT=0]
[Manufacturer]   Xilinx Inc.
[Package]
| variable   typ   min   max
R_pkg   211.500m   205.000m   218.000m
L_pkg   14.500nH   12.200nH   16.800nH
C_pkg   2.150pF   2.000pF   2.300pF
[Pin]  signal_name   model_name   R_pin   L_pin   C_pin
io   iob   IO_100   NA   NA   NA
| End [Component] XCS30XL_PQ240[SLW=1;PCI=0;5VT=0]
|   Component XCS30XL_PQ240[SLW=1;PCI=0;5VT=1]
[Component]   XCS30XL_PQ240[SLW=1;PCI=0;5VT=1]
[Manufacturer]   Xilinx Inc.
[Package]
| variable   typ   min   max
R_pkg   211.500m   205.000m   218.000m
L_pkg   14.500nH   12.200nH   16.800nH
C_pkg   2.150pF   2.000pF   2.300pF
[Pin]  signal_name   model_name   R_pin   L_pin   C_pin
io   iob   IO_101   NA   NA   NA
| End [Component] XCS30XL_PQ240[SLW=1;PCI=0;5VT=1]
|   Component XCS30XL_PQ240[SLW=1;PCI=1;5VT=0]
[Component]   XCS30XL_PQ240[SLW=1;PCI=1;5VT=0]
[Manufacturer]   Xilinx Inc.
[Package]
| variable   typ   min   max
R_pkg   211.500m   205.000m   218.000m
L_pkg   14.500nH   12.200nH   16.800nH
C_pkg   2.150pF   2.000pF   2.300pF
[Pin]  signal_name   model_name   R_pin   L_pin   C_pin
io   iob   IO_110   NA   NA   NA
| End [Component] XCS30XL_PQ240[SLW=1;PCI=1;5VT=0]
|   Component XCS30XL_PQ240[SLW=1;PCI=1;5VT=1]
[Component]   XCS30XL_PQ240[SLW=1;PCI=1;5VT=1]
[Manufacturer]   Xilinx Inc.
[Package]
| variable   typ   min   max
R_pkg   211.500m   205.000m   218.000m
L_pkg   14.500nH   12.200nH   16.800nH
C_pkg   2.150pF   2.000pF   2.300pF
[Pin]  signal_name   model_name   R_pin   L_pin   C_pin
io   iob   IO_111   NA   NA   NA
| End [Component] XCS30XL_PQ240[SLW=1;PCI=1;5VT=1]
|+++++++++++++++++++++++++++++++++++++++++++++++++++++++++++++++++++++++++
|   Component XCS30XL_BG256[SLW=0;PCI=0;5VT=0]
[Component]   XCS30XL_BG256[SLW=0;PCI=0;5VT=0]
[Manufacturer]   Xilinx Inc.
[Package]
| variable   typ   min   max
R_pkg   197.000m   179.000m   215.000m
L_pkg   9.100nH   8.000nH   10.200nH
C_pkg   1.500pF   1.300pF   1.700pF
[Pin]  signal_name   model_name   R_pin   L_pin   C_pin
io   iob   IO_000   NA   NA   NA
| End [Component] XCS30XL_BG256[SLW=0;PCI=0;5VT=0]
|   Component XCS30XL_BG256[SLW=0;PCI=0;5VT=1]
[Component]   XCS30XL_BG256[SLW=0;PCI=0;5VT=1]
[Manufacturer]   Xilinx Inc.
[Package]
| variable   typ   min   max
R_pkg   197.000m   179.000m   215.000m
L_pkg   9.100nH   8.000nH   10.200nH
C_pkg   1.500pF   1.300pF   1.700pF
[Pin]  signal_name   model_name   R_pin   L_pin   C_pin
io   iob   IO_001   NA   NA   NA
| End [Component] XCS30XL_BG256[SLW=0;PCI=0;5VT=1]
|   Component XCS30XL_BG256[SLW=0;PCI=1;5VT=0]
[Component]   XCS30XL_BG256[SLW=0;PCI=1;5VT=0]
[Manufacturer]   Xilinx Inc.
[Package]
| variable   typ   min   max
R_pkg   197.000m   179.000m   215.000m
L_pkg   9.100nH   8.000nH   10.200nH
C_pkg   1.500pF   1.300pF   1.700pF
[Pin]  signal_name   model_name   R_pin   L_pin   C_pin
io   iob   IO_010   NA   NA   NA
| End [Component] XCS30XL_BG256[SLW=0;PCI=1;5VT=0]
|   Component XCS30XL_BG256[SLW=0;PCI=1;5VT=1]
[Component]   XCS30XL_BG256[SLW=0;PCI=1;5VT=1]
[Manufacturer]   Xilinx Inc.
[Package]
| variable   typ   min   max
R_pkg   197.000m   179.000m   215.000m
L_pkg   9.100nH   8.000nH   10.200nH
C_pkg   1.500pF   1.300pF   1.700pF
[Pin]  signal_name   model_name   R_pin   L_pin   C_pin
io   iob   IO_011   NA   NA   NA
| End [Component] XCS30XL_BG256[SLW=0;PCI=1;5VT=1]
|   Component XCS30XL_BG256[SLW=1;PCI=0;5VT=0]
[Component]   XCS30XL_BG256[SLW=1;PCI=0;5VT=0]
[Manufacturer]   Xilinx Inc.
[Package]
| variable   typ   min   max
R_pkg   197.000m   179.000m   215.000m
L_pkg   9.100nH   8.000nH   10.200nH
C_pkg   1.500pF   1.300pF   1.700pF
[Pin]  signal_name   model_name   R_pin   L_pin   C_pin
io   iob   IO_100   NA   NA   NA
| End [Component] XCS30XL_BG256[SLW=1;PCI=0;5VT=0]
|   Component XCS30XL_BG256[SLW=1;PCI=0;5VT=1]
[Component]   XCS30XL_BG256[SLW=1;PCI=0;5VT=1]
[Manufacturer]   Xilinx Inc.
[Package]
| variable   typ   min   max
R_pkg   197.000m   179.000m   215.000m
L_pkg   9.100nH   8.000nH   10.200nH
C_pkg   1.500pF   1.300pF   1.700pF
[Pin]  signal_name   model_name   R_pin   L_pin   C_pin
io   iob   IO_101   NA   NA   NA
| End [Component] XCS30XL_BG256[SLW=1;PCI=0;5VT=1]
|   Component XCS30XL_BG256[SLW=1;PCI=1;5VT=0]
[Component]   XCS30XL_BG256[SLW=1;PCI=1;5VT=0]
[Manufacturer]   Xilinx Inc.
[Package]
| variable   typ   min   max
R_pkg   197.000m   179.000m   215.000m
L_pkg   9.100nH   8.000nH   10.200nH
C_pkg   1.500pF   1.300pF   1.700pF
[Pin]  signal_name   model_name   R_pin   L_pin   C_pin
io   iob   IO_110   NA   NA   NA
| End [Component] XCS30XL_BG256[SLW=1;PCI=1;5VT=0]
|   Component XCS30XL_BG256[SLW=1;PCI=1;5VT=1]
[Component]   XCS30XL_BG256[SLW=1;PCI=1;5VT=1]
[Manufacturer]   Xilinx Inc.
[Package]
| variable   typ   min   max
R_pkg   197.000m   179.000m   215.000m
L_pkg   9.100nH   8.000nH   10.200nH
C_pkg   1.500pF   1.300pF   1.700pF
[Pin]  signal_name   model_name   R_pin   L_pin   C_pin
io   iob   IO_111   NA   NA   NA
| End [Component] XCS30XL_BG256[SLW=1;PCI=1;5VT=1]
|+++++++++++++++++++++++++++++++++++++++++++++++++++++++++++++++++++++++++
|   Component XCS40XL_PQ208[SLW=0;PCI=0;5VT=0]
[Component]   XCS40XL_PQ208[SLW=0;PCI=0;5VT=0]
[Manufacturer]   Xilinx Inc.
[Package]
| variable   typ   min   max
R_pkg   195.500m   195.000m   196.000m
L_pkg   14.200nH   12.500nH   15.900nH
C_pkg   1.800pF   1.600pF   2.000pF
[Pin]  signal_name   model_name   R_pin   L_pin   C_pin
io   iob   IO_000   NA   NA   NA
| End [Component] XCS40XL_PQ208[SLW=0;PCI=0;5VT=0]
|   Component XCS40XL_PQ208[SLW=0;PCI=0;5VT=1]
[Component]   XCS40XL_PQ208[SLW=0;PCI=0;5VT=1]
[Manufacturer]   Xilinx Inc.
[Package]
| variable   typ   min   max
R_pkg   195.500m   195.000m   196.000m
L_pkg   14.200nH   12.500nH   15.900nH
C_pkg   1.800pF   1.600pF   2.000pF
[Pin]  signal_name   model_name   R_pin   L_pin   C_pin
io   iob   IO_001   NA   NA   NA
| End [Component] XCS40XL_PQ208[SLW=0;PCI=0;5VT=1]
|   Component XCS40XL_PQ208[SLW=0;PCI=1;5VT=0]
[Component]   XCS40XL_PQ208[SLW=0;PCI=1;5VT=0]
[Manufacturer]   Xilinx Inc.
[Package]
| variable   typ   min   max
R_pkg   195.500m   195.000m   196.000m
L_pkg   14.200nH   12.500nH   15.900nH
C_pkg   1.800pF   1.600pF   2.000pF
[Pin]  signal_name   model_name   R_pin   L_pin   C_pin
io   iob   IO_010   NA   NA   NA
| End [Component] XCS40XL_PQ208[SLW=0;PCI=1;5VT=0]
|   Component XCS40XL_PQ208[SLW=0;PCI=1;5VT=1]
[Component]   XCS40XL_PQ208[SLW=0;PCI=1;5VT=1]
[Manufacturer]   Xilinx Inc.
[Package]
| variable   typ   min   max
R_pkg   195.500m   195.000m   196.000m
L_pkg   14.200nH   12.500nH   15.900nH
C_pkg   1.800pF   1.600pF   2.000pF
[Pin]  signal_name   model_name   R_pin   L_pin   C_pin
io   iob   IO_011   NA   NA   NA
| End [Component] XCS40XL_PQ208[SLW=0;PCI=1;5VT=1]
|   Component XCS40XL_PQ208[SLW=1;PCI=0;5VT=0]
[Component]   XCS40XL_PQ208[SLW=1;PCI=0;5VT=0]
[Manufacturer]   Xilinx Inc.
[Package]
| variable   typ   min   max
R_pkg   195.500m   195.000m   196.000m
L_pkg   14.200nH   12.500nH   15.900nH
C_pkg   1.800pF   1.600pF   2.000pF
[Pin]  signal_name   model_name   R_pin   L_pin   C_pin
io   iob   IO_100   NA   NA   NA
| End [Component] XCS40XL_PQ208[SLW=1;PCI=0;5VT=0]
|   Component XCS40XL_PQ208[SLW=1;PCI=0;5VT=1]
[Component]   XCS40XL_PQ208[SLW=1;PCI=0;5VT=1]
[Manufacturer]   Xilinx Inc.
[Package]
| variable   typ   min   max
R_pkg   195.500m   195.000m   196.000m
L_pkg   14.200nH   12.500nH   15.900nH
C_pkg   1.800pF   1.600pF   2.000pF
[Pin]  signal_name   model_name   R_pin   L_pin   C_pin
io   iob   IO_101   NA   NA   NA
| End [Component] XCS40XL_PQ208[SLW=1;PCI=0;5VT=1]
|   Component XCS40XL_PQ208[SLW=1;PCI=1;5VT=0]
[Component]   XCS40XL_PQ208[SLW=1;PCI=1;5VT=0]
[Manufacturer]   Xilinx Inc.
[Package]
| variable   typ   min   max
R_pkg   195.500m   195.000m   196.000m
L_pkg   14.200nH   12.500nH   15.900nH
C_pkg   1.800pF   1.600pF   2.000pF
[Pin]  signal_name   model_name   R_pin   L_pin   C_pin
io   iob   IO_110   NA   NA   NA
| End [Component] XCS40XL_PQ208[SLW=1;PCI=1;5VT=0]
|   Component XCS40XL_PQ208[SLW=1;PCI=1;5VT=1]
[Component]   XCS40XL_PQ208[SLW=1;PCI=1;5VT=1]
[Manufacturer]   Xilinx Inc.
[Package]
| variable   typ   min   max
R_pkg   195.500m   195.000m   196.000m
L_pkg   14.200nH   12.500nH   15.900nH
C_pkg   1.800pF   1.600pF   2.000pF
[Pin]  signal_name   model_name   R_pin   L_pin   C_pin
io   iob   IO_111   NA   NA   NA
| End [Component] XCS40XL_PQ208[SLW=1;PCI=1;5VT=1]
|+++++++++++++++++++++++++++++++++++++++++++++++++++++++++++++++++++++++++
|   Component XCS40XL_PQ240[SLW=0;PCI=0;5VT=0]
[Component]   XCS40XL_PQ240[SLW=0;PCI=0;5VT=0]
[Manufacturer]   Xilinx Inc.
[Package]
| variable   typ   min   max
R_pkg   211.500m   205.000m   218.000m
L_pkg   14.500nH   12.200nH   16.800nH
C_pkg   2.150pF   2.000pF   2.300pF
[Pin]  signal_name   model_name   R_pin   L_pin   C_pin
io   iob   IO_000   NA   NA   NA
| End [Component] XCS40XL_PQ240[SLW=0;PCI=0;5VT=0]
|   Component XCS40XL_PQ240[SLW=0;PCI=0;5VT=1]
[Component]   XCS40XL_PQ240[SLW=0;PCI=0;5VT=1]
[Manufacturer]   Xilinx Inc.
[Package]
| variable   typ   min   max
R_pkg   211.500m   205.000m   218.000m
L_pkg   14.500nH   12.200nH   16.800nH
C_pkg   2.150pF   2.000pF   2.300pF
[Pin]  signal_name   model_name   R_pin   L_pin   C_pin
io   iob   IO_001   NA   NA   NA
| End [Component] XCS40XL_PQ240[SLW=0;PCI=0;5VT=1]
|   Component XCS40XL_PQ240[SLW=0;PCI=1;5VT=0]
[Component]   XCS40XL_PQ240[SLW=0;PCI=1;5VT=0]
[Manufacturer]   Xilinx Inc.
[Package]
| variable   typ   min   max
R_pkg   211.500m   205.000m   218.000m
L_pkg   14.500nH   12.200nH   16.800nH
C_pkg   2.150pF   2.000pF   2.300pF
[Pin]  signal_name   model_name   R_pin   L_pin   C_pin
io   iob   IO_010   NA   NA   NA
| End [Component] XCS40XL_PQ240[SLW=0;PCI=1;5VT=0]
|   Component XCS40XL_PQ240[SLW=0;PCI=1;5VT=1]
[Component]   XCS40XL_PQ240[SLW=0;PCI=1;5VT=1]
[Manufacturer]   Xilinx Inc.
[Package]
| variable   typ   min   max
R_pkg   211.500m   205.000m   218.000m
L_pkg   14.500nH   12.200nH   16.800nH
C_pkg   2.150pF   2.000pF   2.300pF
[Pin]  signal_name   model_name   R_pin   L_pin   C_pin
io   iob   IO_011   NA   NA   NA
| End [Component] XCS40XL_PQ240[SLW=0;PCI=1;5VT=1]
|   Component XCS40XL_PQ240[SLW=1;PCI=0;5VT=0]
[Component]   XCS40XL_PQ240[SLW=1;PCI=0;5VT=0]
[Manufacturer]   Xilinx Inc.
[Package]
| variable   typ   min   max
R_pkg   211.500m   205.000m   218.000m
L_pkg   14.500nH   12.200nH   16.800nH
C_pkg   2.150pF   2.000pF   2.300pF
[Pin]  signal_name   model_name   R_pin   L_pin   C_pin
io   iob   IO_100   NA   NA   NA
| End [Component] XCS40XL_PQ240[SLW=1;PCI=0;5VT=0]
|   Component XCS40XL_PQ240[SLW=1;PCI=0;5VT=1]
[Component]   XCS40XL_PQ240[SLW=1;PCI=0;5VT=1]
[Manufacturer]   Xilinx Inc.
[Package]
| variable   typ   min   max
R_pkg   211.500m   205.000m   218.000m
L_pkg   14.500nH   12.200nH   16.800nH
C_pkg   2.150pF   2.000pF   2.300pF
[Pin]  signal_name   model_name   R_pin   L_pin   C_pin
io   iob   IO_101   NA   NA   NA
| End [Component] XCS40XL_PQ240[SLW=1;PCI=0;5VT=1]
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| Models and submodels in the file (8): IO_000 (I/O), IO_001 (I/O), IO_010 (I/O), IO_011 (I/O), IO_100 (I/O), IO_101 (I/O), IO_110 (I/O), IO_111 (I/O)
